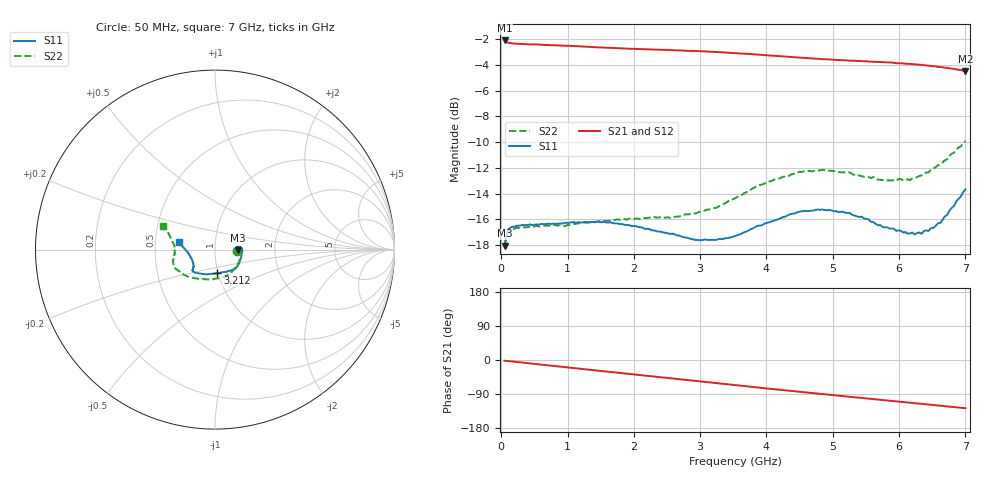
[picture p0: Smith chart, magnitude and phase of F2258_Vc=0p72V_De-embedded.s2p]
! Integrated Device Technology
! Corporate Headquarters
! 6024 Silver Creek Valley Road
! San Jose, CA 95138  USA
! Phone:  1-408-284-8200
! Toll Free:  1-800-223-1366
! Webpage:  http://www.idt.com/
! Timing and RF Division
! 515 Groton Road, Suite 102
! Westford, MA 01886-6024
! Device:  F2258
! Description: Voltage Variable RF Attenuator
! Frequency:  50.0 -  6000.00 MHz
! Package:  3x3 mm Thin QFN Plastic Package: 16 pin
! Ports:  2 RF, 2 DC
!  Pin  1  = NC
!  Pin  2  = NC
!  Pin  3  = RF2  = Port 2
!  Pin  4  = GND
!  Pin  5  = Vdd
!  Pin  6  = NC
!  Pin  7  = VCTRL
!  Pin  8  = NC
!  Pin  9  = GND
!  Pin 10  = RF1  = Port 1
!  Pin 11  = NC
!  Pin 12  = NC
!  Pin 13  = NC
!  Pin 14  = NC
!  Pin 15  = NC
!  Pin 16  = NC
! Vcntrl:  0.720 Volts
! Vdd:  +3.300 Volts
! Current:  1.122 mA
! Data:  The device was measured on a the F2258 evaluation board which has
!  individual transmission lines to the RF pins.  Data was collected
!  using a calibrated network analyzer.  The evaluation board was
!  de-embedded using a TRL calibration technique.
!  The reference plane is the edge of the package pin.
! Misc:  SN 10
!  Action Tracker AT0285
! Date Measured:  2014-12-10
! Date:  2016-01-13  MJV
! Note:
!  Integrated Device Technology supplies this data as a sample of measured
!  data at the package pin for this product.  Your particular data for this
!  product may vary.
!  Data was taken at 25 degrees C.
!  Integrated Device Technology reserves the right to change this data at anytime.
!Freq_(GHz)  S11M_(dB)  S11P_(deg)  S21M_(dB)  S21P_(deg)  S12M_(dB)  S12P_(deg)  S22M_(dB)  S22P_(deg)
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# GHz S dB R 50
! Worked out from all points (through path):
!   201 points, 50 MHz to 7 GHz, reference 50 ohm
!   highest |S21| = -2.10 dB at 50 MHz (marker M1); lowest = -4.5 dB at 7 GHz (marker M2)
!   group delay of S21, straight-line fit = 50.3 ps
!   lowest |S11| = -18.0 dB at 50 MHz (marker M3), VSWR 1.29, Z = 64.3 - j0.504 ohm
!   |S11| at or under -10 dB: start of sweep to end of sweep
!   |S22| runs from -18.1 to -9.9 dB; largest |S21 - S12| = 0.0014
!   S11 on the Smith chart (normalised r, x): 50 MHz: 1.29, -0.01; 3.212 GHz: 0.99, -0.26; 7 GHz: 0.66, +0.06
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0.05  -18.03 -1.8  -2.10 -2.0  -2.10 -2.0  -18.07 -2.6
0.08475  -17.01 -2.8  -2.24 -2.5  -2.23 -2.5  -17.12 -3.8
0.15425  -16.58 -4.6  -2.32 -3.7  -2.31 -3.7  -16.75 -6.7
0.71025  -16.32 -21.0  -2.46 -14.2  -2.45 -14.2  -16.47 -28.3
0.9535  -16.25 -28.8  -2.50 -18.8  -2.50 -18.8  -16.52 -38.5
1.2315  -16.23 -35.3  -2.57 -23.9  -2.57 -23.9  -16.27 -48.2
1.6485  -16.21 -43.5  -2.67 -31.5  -2.67 -31.5  -16.07 -61.0
2.37825  -16.94 -56.6  -2.82 -44.7  -2.81 -44.7  -15.84 -80.9
2.58675  -17.10 -61.7  -2.85 -48.6  -2.85 -48.6  -15.87 -87.4
2.93425  -17.59 -72.9  -2.92 -55.0  -2.93 -55.0  -15.53 -99.7
3.21225  -17.59 -84.3  -2.99 -60.3  -2.98 -60.3  -15.11 -110.8
3.525  -17.28 -98.3  -3.08 -66.2  -3.08 -66.2  -14.35 -123.3
4.0115  -16.25 -118.4  -3.25 -75.2  -3.26 -75.2  -13.08 -140.4
4.46325  -15.43 -130.2  -3.42 -83.4  -3.42 -83.4  -12.35 -152.6
4.7065  -15.31 -133.5  -3.50 -87.6  -3.50 -87.6  -12.24 -157.3
5.2625  -15.51 -138.6  -3.67 -97.2  -3.67 -97.2  -12.35 -166.5
5.85325  -16.71 -145.1  -3.81 -107.4  -3.82 -107.4  -12.96 -177.7
6.166  -17.08 -152.9  -3.92 -112.9  -3.91 -112.9  -12.94 175.4
6.2355  -17.17 -156.4  -3.96 -114.0  -3.95 -114.1  -12.76 173.4
6.444  -16.88 -166.0  -4.05 -117.8  -4.06 -117.8  -12.34 168.4
6.61775  -16.27 -175.7  -4.16 -120.8  -4.17 -120.8  -11.72 163.7
7  -13.66 168.4  -4.47 -127.1  -4.47 -127.1  -9.91 155.5
